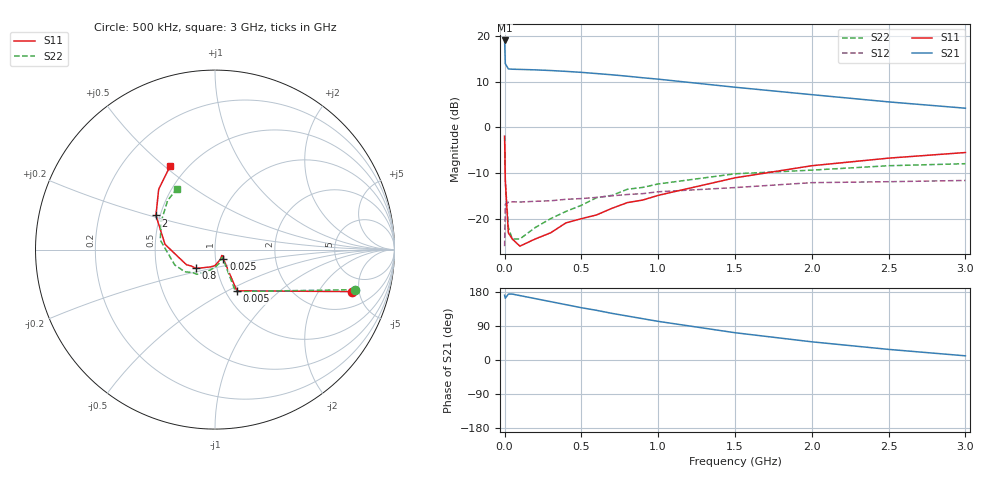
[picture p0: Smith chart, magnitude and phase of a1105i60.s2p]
!  MSA-1105 S AND NOISE PARAMETERS
!  Id=60mA  LAST UPDATED 07-27-92
# ghz s ma r 50
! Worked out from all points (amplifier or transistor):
!   18 points, 500 kHz to 3 GHz, reference 50 ohm
!   highest |S21| = 19.0 dB at 500 kHz (marker M1)
!   |S21| within 3 dB of that: start of sweep to 3.156 MHz
!   unconditionally stable (mu >= 1): 11.42 MHz to 998.5 MHz; 1.24 GHz to 1.514 GHz; 2.184 GHz to end of sweep
!   at 50 MHz: K = 1.08, MAG = 12.8 dB, |S12| = -16.3 dB
!   at 600 MHz: K = 1.04, MAG = 12.4 dB, |S12| = -15.3 dB
!   at 3 GHz: K = 1.04, MAG = 6.7 dB, |S12| = -11.6 dB
!   lowest NFmin = 3.40 dB at 100 MHz
!   S11 on the Smith chart (normalised r, x): 500 kHz: 3.28, -4.26; 5 MHz: 1.13, -0.56; 25 MHz: 1.09, -0.11; 800 MHz: 0.79, -0.17; 2 GHz: 0.47, +0.21; 3 GHz: 0.40, +0.53
0.0005  0.8 -17.0  8.94 171.0  0.05 51.0  0.81 -16.0
0.005  0.26 -62.0  4.98 163.0  0.144 15.0  0.26 -64.0
0.025  0.07 -48.0  4.36 174.0  0.151 4.0  0.08 -52.0
0.05  0.06 -38.0  4.33 174.0  0.153 2.0  0.06 -48.0
0.1  0.05 -41.0  4.31 170.0  0.152 3.0  0.06 -52.0
0.2  0.06 -58.0  4.26 162.0  0.155 5.0  0.08 -73.0
0.3  0.07 -74.0  4.19 154.0  0.157 7.0  0.1 -91.0
0.4  0.09 -91.0  4.1 146.0  0.163 8.0  0.12 -105.0
0.5  0.1 -105.0  4 138.0  0.166 8.0  0.14 -116.0
0.6  0.11 -116.0  3.88 131.0  0.171 10.0  0.17 -126.0
0.7  0.13 -128.0  3.76 123.0  0.178 11.0  0.18 -135.0
0.8  0.15 -136.0  3.63 116.0  0.184 11.0  0.21 -144.0
0.9  0.16 -145.0  3.49 109.0  0.188 11.0  0.22 -151.0
1  0.18 -152.0  3.37 102.0  0.197 11.0  0.24 -159.0
1.5  0.28 174.0  2.75 72.0  0.219 7.0  0.31 170.0
2  0.38 150.0  2.28 48.0  0.248 0.0  0.34 151.0
2.5  0.46 133.0  1.9 28.0  0.254 -4.0  0.38 134.0
3  0.53 118.0  1.62 11.0  0.262 -8.0  0.4 122.0
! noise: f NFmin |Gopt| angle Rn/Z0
0.1  3.4  0.02  8  0.43
0.5  3.6  0.02  106  0.42
1  4.1  0.05  179  0.41
2  5.4  0.18  -132  0.44
